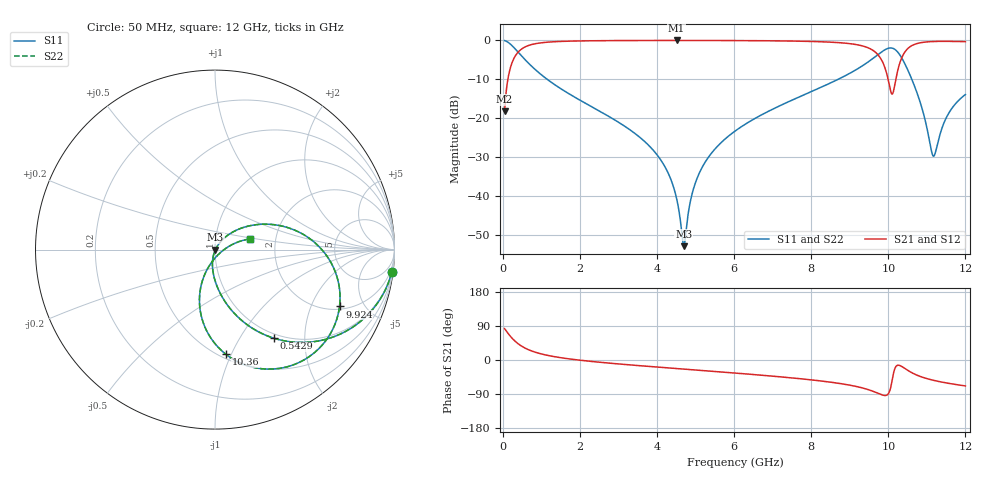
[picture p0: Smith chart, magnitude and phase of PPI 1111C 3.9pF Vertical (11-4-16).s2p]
# GHz S MA R 50
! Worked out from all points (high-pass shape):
!   1601 points, 50 MHz to 12 GHz, reference 50 ohm
!   highest |S21| = -0.02 dB at 4.509 GHz (marker M1); lowest = -18.2 dB at 50 MHz (marker M2)
!   |S21| within 3 dB of the highest: 400.1 MHz to 9.665 GHz (9.265 GHz wide, 184 % of centre); 10.43 GHz to end of sweep
!   lowest |S11| = -52.8 dB at 4.696 GHz (marker M3), VSWR 1.00, Z = 50.2 - j0.103 ohm
!   |S11| at or under -10 dB: 1.155 GHz to 8.698 GHz (7.542 GHz wide, 153 % of centre); 10.61 GHz to end of sweep
!   |S22| runs from -52.8 to -0.1 dB; largest |S21 - S12| = 0
!   S11 on the Smith chart (normalised r, x): 50 MHz: 1, -16; 542.9 MHz: 0.93, -1.42; 9.924 GHz: 2.16, -3.26; 10.36 GHz: 0.54, -0.95; 12 GHz: 1.47, +0.18
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0.05  0.9924 -7.3  0.1232 82.7  0.1232 82.7  0.9924 -7.3
0.22925  0.8686 -30.9  0.4952 59.1  0.4952 59.1  0.8686 -30.9
0.5429375  0.5919 -56.5  0.8053 33.5  0.8053 33.5  0.5919 -56.5
1.058281  0.3442 -75.2  0.9378 14.6  0.9378 14.6  0.3442 -75.2
2.044156  0.1666 -90.5  0.9845 -1.0  0.9845 -1.0  0.1666 -90.5
4.038312  0.03231 -105.3  0.9972 -18.9  0.9972 -18.9  0.03231 -105.3
4.508844  0.009439 -99.0  0.9975 -22.6  0.9975 -22.6  0.009439 -99.0
4.695563  0.002294 -26.6  0.9974 -24.0  0.9974 -24.0  0.002294 -26.6
4.904687  0.01038 51.1  0.9973 -25.6  0.9973 -25.6  0.01038 51.1
5.121281  0.02095 55.9  0.997 -27.3  0.997 -27.3  0.02095 55.9
6.025  0.06857 53.1  0.9943 -34.4  0.9943 -34.4  0.06857 53.1
8.019156  0.2219 35.7  0.9683 -52.6  0.9683 -52.6  0.2219 35.7
9.378469  0.4894 10.7  0.8361 -75.1  0.8361 -75.1  0.4894 10.7
9.684688  0.6296 -3.9  0.692 -85.7  0.692 -85.7  0.6296 -3.9
9.923687  0.7626 -24.5  0.4295 -93.7  0.4295 -93.7  0.7626 -24.5
10.01331  0.7947 -35.5  0.2881 -87.1  0.2881 -87.1  0.7947 -35.5
10.12534  0.7886 -51.5  0.2144 -39.9  0.2144 -39.9  0.7886 -51.5
10.35688  0.5859 -84.1  0.6099 -17.5  0.6099 -17.5  0.5859 -84.1
10.79753  0.1785 -112.2  0.9242 -42.2  0.9242 -42.2  0.1785 -112.2
11.17097  0.03269 -48.7  0.9669 -53.6  0.9669 -53.6  0.03269 -48.7
11.53694  0.1094 17.3  0.9716 -61.1  0.9716 -61.1  0.1094 17.3
12  0.2023 17.0  0.9627 -68.4  0.9627 -68.4  0.2023 17.0
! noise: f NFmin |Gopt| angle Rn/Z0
0.05  0.000457  0.9087  2.848  0.0011
1.372  0.00393  0.6872  8.262  0.002428
2.701  0.006481  0.6397  14.62  0.003343
4.031  0.008879  0.6182  20.92  0.004198
5.36  0.01144  0.6147  27.03  0.005234
6.682  0.01475  0.6327  32.93  0.006972
8.012  0.02133  0.6937  38.87  0.01213
9.341  0.05471  0.8526  45.27  0.06753
10.67  0.08825  0.8967  51.45  0.1515
12  0.03936  0.7666  56.36  0.02679
